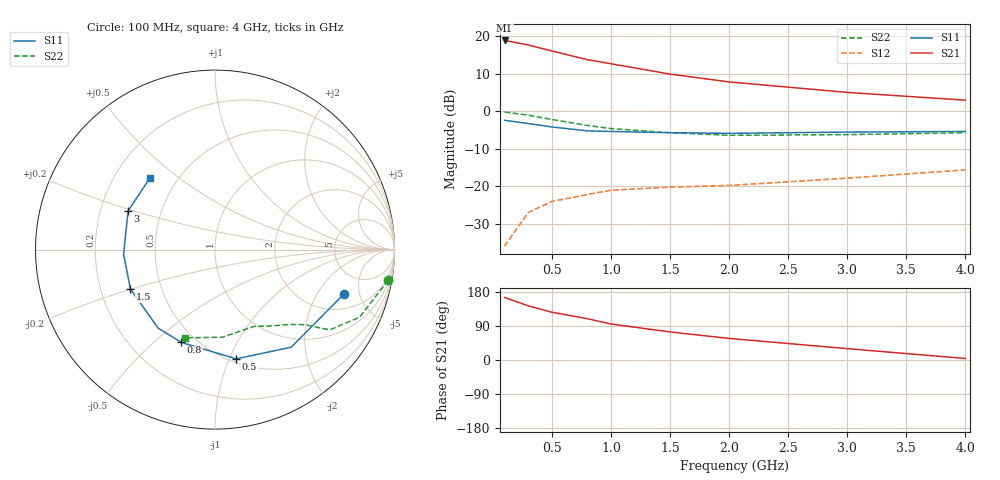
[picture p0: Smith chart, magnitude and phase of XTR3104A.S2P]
! HXTR-3104  (2N6839) Common Emitter
! Vce=15V  Ic=20mA
# ghz s ma r 50
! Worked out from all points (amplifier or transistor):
!   9 points, 100 MHz to 4 GHz, reference 50 ohm
!   highest |S21| = 18.9 dB at 100 MHz (marker M1)
!   |S21| within 3 dB of that: start of sweep to 525.6 MHz
!   unconditionally stable (mu >= 1): 1.905 GHz to 3.446 GHz
!   at 300 MHz: K = 0.22, MSG = 22.3 dB, |S12| = -26.9 dB
!   at 1 GHz: K = 0.63, MSG = 16.9 dB, |S12| = -21.0 dB
!   at 4 GHz: K = 0.94, MSG = 9.3 dB, |S12| = -15.6 dB
!   S11 on the Smith chart (normalised r, x): 100 MHz: 3.01, -3.52; 500 MHz: 0.54, -1.06; 800 MHz: 0.42, -0.62; 1.5 GHz: 0.33, -0.20; 3 GHz: 0.32, +0.19; 4 GHz: 0.35, +0.40
0.1  0.76 -19.0  8.81 165.0  0.016 72.0  0.98 -10.0
0.3  0.69 -52.0  7.67 143.0  0.045 60.0  0.89 -25.0
0.5  0.62 -79.0  6.38 126.0  0.063 50.0  0.78 -35.0
0.8  0.55 -110.0  4.89 109.0  0.078 41.0  0.65 -40.0
1  0.54 -126.0  4.31 95.0  0.089 34.0  0.59 -45.0
1.5  0.52 -155.0  3.14 74.0  0.098 30.0  0.52 -55.0
2  0.51 -177.0  2.47 57.0  0.103 29.0  0.48 -63.0
3  0.53 156.0  1.79 30.0  0.129 31.0  0.49 -85.0
4  0.54 132.0  1.41 4.0  0.166 29.0  0.52 -109.0
